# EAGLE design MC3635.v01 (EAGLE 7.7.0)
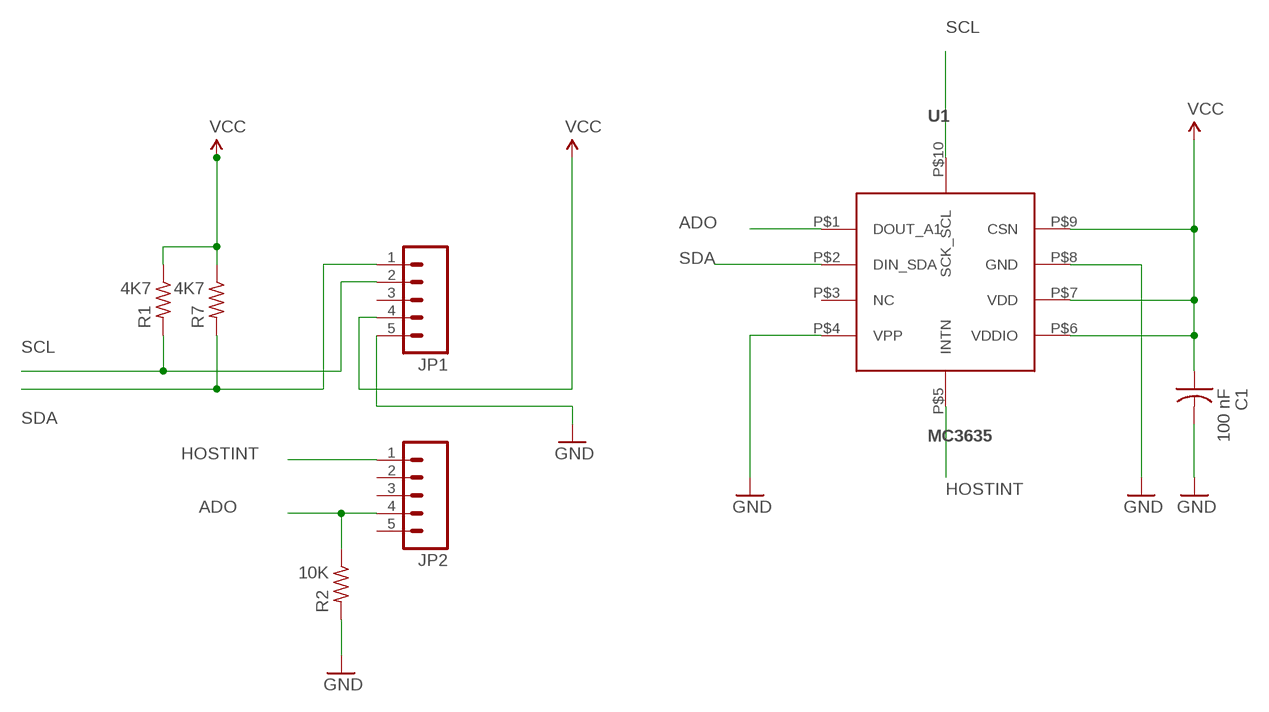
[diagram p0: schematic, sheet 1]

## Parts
C1  100 nF  C-US  [C0402_B]
JP1  M05NO_SILK  [1X05_NO_SILK]
JP2  M05NO_SILK  [1X05_NO_SILK]
R1  4K7  R-US_  [R0402_B]
R2  10K  R-US_  [R0402_B]
R7  4K7  R-US_  [R0402_B]
U1  MC3635  [MC3635]

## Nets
ADO: JP2.4 R2.1 U1.P$1(DOUT_A1)
GND: C1.2 JP1.5 R2.2 U1.P$4(VPP) U1.P$8(GND)
HOSTINT: JP2.1 U1.P$5(INTN)
SCL: JP1.2 R1.2 U1.P$10(SCK_SCL)
SDA: JP1.1 R7.2 U1.P$2(DIN_SDA)
VCC: C1.1 JP1.4 R1.1 R7.1 U1.P$6(VDDIO) U1.P$7(VDD) U1.P$9(CSN)
Unconnected: JP1.3 JP2.2 JP2.3 JP2.5 U1.P$3(NC)

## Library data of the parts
C1 = Spark:C-US: Capacitor
JP1 JP2 = SparkFun-Connectors:M05: Header 5 Standard 5-pin 0.1" header. Use with straight break away headers (SKU : PRT-00116), right angle break away headers (PRT-00553), swiss pins (PRT-00743), machine pins (PRT-00117), and female headers (PRT-00115). Molex polarized connector foot print use with SKU : PRT-08230 with associated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
R1 R2 R7 = Spark:R-US_: 0402 Resistor
U1 = kris:MC3635: MEMSIC MC3635 utra-low-power 3-axis accelerometer https://www.mouser.com/pdfDocs/MEMSIC_MC3635_Datasheet.pdf

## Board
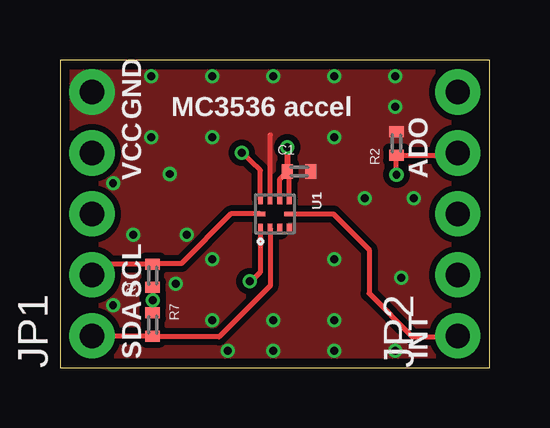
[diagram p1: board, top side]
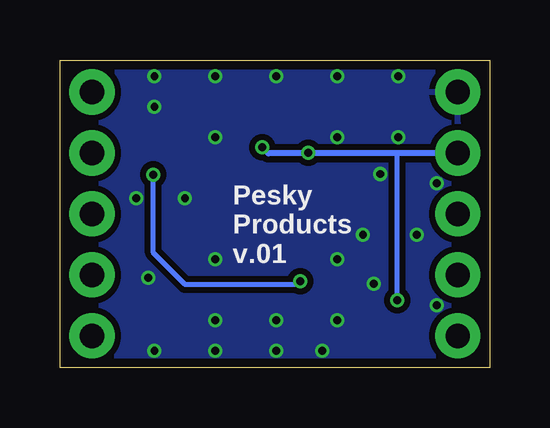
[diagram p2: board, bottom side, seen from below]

Size 17.91 x 12.83 mm. Coordinates in mm from the lower left corner, seen from the top.
Outline: 0,0 17.91,0 17.91,12.83 0,12.83 0,0
Copper layers (1*16): Top 0.035559375mm / dielectric 1.6mm / Bottom 0.035559375mm
Design rules "oshpark-2layer *": minimum track width 6mil, minimum drill 10mil, track to track 6mil, track to pad 6mil, pad to pad 6mil, via to via 6mil, smd to smd 6mil, copper to edge 15mil, drill to drill 6mil, minimum pad ring 5mil, minimum via ring 5mil, stop-mask expansion 2.5mil, vias tented up to drill 20mil, thermal gap 10mil

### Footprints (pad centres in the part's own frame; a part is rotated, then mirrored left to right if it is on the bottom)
C0402_B = smd 0.457 x 0.61: 1 -0.483,0; 2 0.483,0
1X05_NO_SILK = drill 1.016 pad 1.88: 1 0,0; 2 2.54,0; 3 5.08,0; 4 7.62,0; 5 10.16,0
R0402_B = smd 0.457 x 0.61: 1 -0.483,0; 2 0.483,0
MC3635 = smd 0.4 x 0.2: P$1 0.6,-0.6; P$2 0.6,-0.2; P$3 0.6,0.2; P$4 0.6,0.6; P$6 -0.6,0.6; P$7 -0.6,0.2; P$8 -0.6,-0.2; P$9 -0.6,-0.6 | smd 0.2 x 0.4: P$5 0,0.6; P$10 0,-0.6

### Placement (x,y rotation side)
C1  9.96,8.18 0 top
JP1  1.33,1.33 90 top
JP2  16.57,1.33 90 top
R1  3.86,3.84 90 top
R2  14.02,9.35 90 top
R7  3.86,1.8 270 top
U1  8.95,6.41 270 top

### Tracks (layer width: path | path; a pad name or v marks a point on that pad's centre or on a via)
ADO  (via drill 0.33)
  Top 0.203: U1.P$1 8.35,3.98 7.98,3.61 v7.9,3.61 | v14.02,8.05 R2.1 16.43,8.87 JP2.4
  Bottom 0.203: v14.02,8.05 14.02,4.8 12.7,3.48 7.77,3.48 v7.9,3.61
GND  (via drill 0.33)
  Top 0.203: U1.P$8 8.75,9.69 8.76,9.7
  other vias: 3.81,12.14 6.35,12.14 8.89,12.14 11.43,12.14 13.97,12.14 11.43,9.6 6.35,9.6 3.81,9.6 5.28,5.54 12.7,7.06 11.43,1.98 8.89,1.98 6.35,1.98 6.35,4.52 11.43,4.52 3.05,5.54 14.22,3.76 4.57,8.08 4.83,3.51 14.73,7.06 13.97,10.87 13.97,0.71 11.43,0.71 8.89,0.71 6.99,0.71 2.21,2.62 2.21,7.7
  pour Bottom (isolate 0.254): 0,12.83 17.91,12.83 17.91,0 0,0
  pour Top (isolate 0.254, no thermals): 0,12.83 17.91,12.83 17.91,0 0,0
HOSTINT
  Top 0.203: U1.P$5 11.39,6.41 12.88,4.93 12.88,3.1 14.68,1.29 16.54,1.29 JP2.1
SCL
  Top 0.203: JP1.2 1.78,4.32 R1.2 3.89,4.34 5.05,4.34 7.12,6.41 U1.P$10
SDA
  Top 0.203: U1.P$2 8.75,3.42 6.63,1.29 3.89,1.29 R7.2 1.35,1.32 JP1.1
VCC  (via drill 0.33)
  Top 0.203: R1.1 v3.86,2.82 R7.1 | U1.P$7 9.15,7.86 C1.1 9.55,8.1 U1.P$6 | U1.P$9 8.35,8.23 v7.57,8.97
  Top 0.254: v9.47,9.2 C1.1
  Bottom 0.203: v3.86,2.82 3.86,8.91 3.83,8.94 | v7.57,8.97 7.57,9.07 7.7,8.94
  Bottom 0.254: v9.47,9.2 9.22,8.94 7.7,8.94 3.83,8.94 1.35,8.94 JP1.4

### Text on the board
tPlace: GND | MC3536 accel | VCC | ADO | SCL | SDA | INT
bPlace: Pesky / Products / v.01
